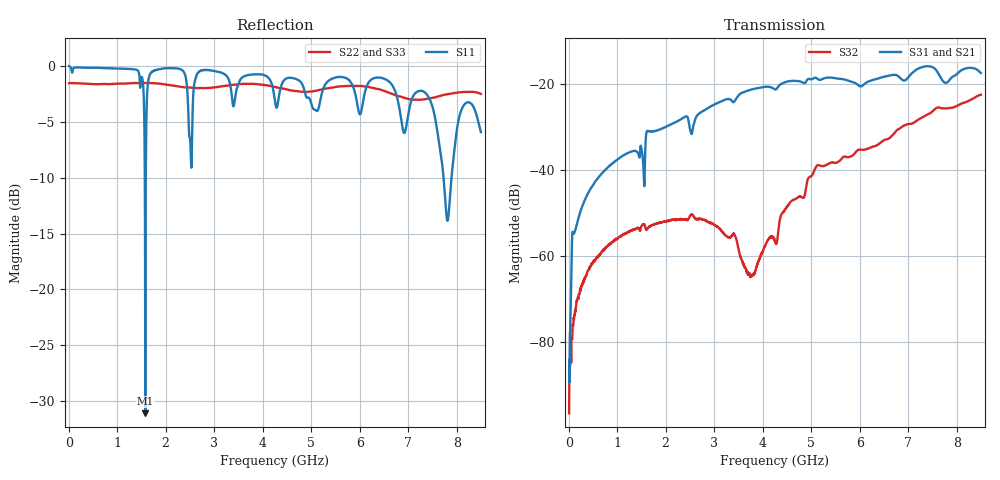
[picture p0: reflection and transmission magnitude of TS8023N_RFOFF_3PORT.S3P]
!Agilent Technologies,E5071C,MY46522130,B.12.04
!Date: Thu Jul 17 20:33:02 2025
!Data & Calibration Information:
!Freq	S11:SOLT3(ON)	S13:SOLT3(ON)	S14:SOLT3(ON)
!	S31:SOLT3(ON)	S33:SOLT3(ON)	S34:SOLT3(ON)
!	S41:SOLT3(ON)	S43:SOLT3(ON)	S44:SOLT3(ON)
!PortZ  Port1:50+j0  Port3:50+j0  Port4:50+j0
!Above PortZ is port z conversion or system Z0 setting when saving the data.
!When reading, reference impedance value at option line is always used.
# Hz S dB R 50
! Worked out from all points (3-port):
!   1601 points, 10 MHz to 8.5 GHz, reference 50 ohm
!   strongest paths, dB at 10 MHz, 2.132 GHz, 4.255 GHz, 6.378 GHz, 8.5 GHz:
!     S31: -84.1, -29.2, -21.2, -18.7, -17.4
!     S21: -87.0, -29.4, -21.4, -19.0, -17.8
!     S32: -96.5, -51.5, -56.4, -34.0, -22.4
!   lowest |S11| = -31.1 dB at 1.581 GHz (marker M1), VSWR 1.06, Z = 49 + j2.57 ohm
!   |S11| at or under -10 dB: 1.57 GHz to 1.591 GHz (20.33 MHz wide, 1.29 % of centre); 7.73 GHz to 7.894 GHz (164 MHz wide, 2.1 % of centre)
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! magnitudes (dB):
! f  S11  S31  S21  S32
! 10 MHz  0.0  -84.1  -87.0  -96.5
! 105.5 MHz  -0.2  -54.7  -54.8  -74.2
! 323.1 MHz  -0.1  -47.2  -47.3  -65.1
! 1.581 GHz  -31.1  -35.1  -35.6  -53.3
! 2.812 GHz  -0.3  -26.0  -26.0  -51.6
! 3.772 GHz  -0.8  -21.2  -21.5  -64.6
! 4.255 GHz  -3.1  -21.2  -21.4  -56.4
! 5.131 GHz  -4.0  -18.8  -18.8  -38.8
! 7.81 GHz  -13.9  -19.6  -19.5  -25.6
! 8.5 GHz  -5.9  -17.4  -17.8  -22.4
